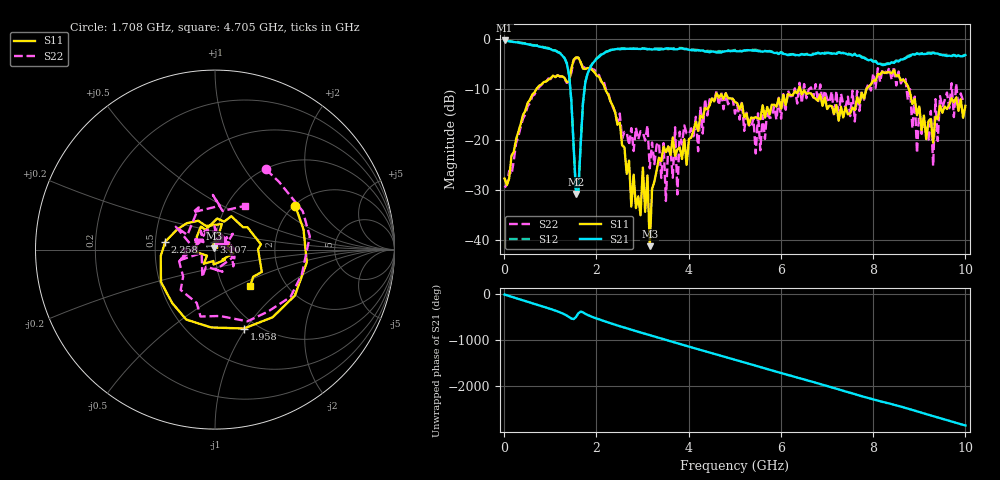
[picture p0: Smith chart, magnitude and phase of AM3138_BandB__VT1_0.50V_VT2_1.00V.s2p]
! Date/Time: Tue, Nov 13, 2018 4:39 PM
! Network Analyzer: Agilent Technologies E8364B Rev: A.07.50.67
! Sweep from 0.010 to 10.000 GHz, 201 Points, Sweep Type: LIN
! Power Supply: 0.500 V, 0.000 A
# Hz S DB R 50
!freq MagS11 AngS11 MagS21 AngS21 MagS12 AngS12 MagS22 AngS22
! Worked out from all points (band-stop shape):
!   201 points, 10 MHz to 10 GHz, reference 50 ohm
!   highest |S21| = -0.24 dB at 10 MHz (marker M1); lowest = -30.9 dB at 1.558 GHz (marker M2)
!   |S21| within 3 dB of the highest: start of sweep to 1.258 GHz; 2.091 GHz to 7.641 GHz (5.55 GHz wide, 114 % of centre)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
!   lowest |S11| = -41.3 dB at 3.157 GHz (marker M3), VSWR 1.02, Z = 49.6 + j0.782 ohm
!   |S11| at or under -10 dB: 2.195 GHz to 6.383 GHz (4.189 GHz wide, 97.7 % of centre); 6.421 GHz to 7.852 GHz (1.431 GHz wide, 20 % of centre); 8.777 GHz to end of sweep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
!   |S22| runs from -32.3 to -3.7 dB; largest |S21 - S12| = 0.028
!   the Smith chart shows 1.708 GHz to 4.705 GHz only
!   S11 on the Smith chart (normalised r, x): 1.708 GHz: 2.03, +1.33; 1.958 GHz: 0.87, -0.98; 2.258 GHz: 0.56, +0.05; 3.107 GHz: 0.98, +0.08; 4.705 GHz: 1.33, -0.60
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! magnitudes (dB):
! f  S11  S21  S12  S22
! 10 MHz  -27.8  -0.2  -0.3  -29.6
! 1.309 GHz  -7.7  -3.8  -3.7  -7.9
! 1.558 GHz  -3.6  -30.9  -30.7  -3.8
! 1.708 GHz  -5.9  -12.8  -12.8  -5.5
! 1.958 GHz  -6.6  -4.4  -4.3  -6.1
! 2.258 GHz  -11.0  -2.4  -2.4  -10.6
! 2.757 GHz  -33.4  -1.9  -1.9  -17.7
! 3.107 GHz  -27.2  -1.9  -2.0  -17.2
! 3.157 GHz  -41.3  -2.0  -1.9  -25.7
! 3.357 GHz  -23.6  -2.1  -1.8  -20.6
! 3.507 GHz  -22.5  -1.8  -1.9  -32.3
! 3.706 GHz  -23.3  -2.0  -1.8  -17.5
! 3.756 GHz  -22.0  -2.0  -1.8  -30.9
! 3.806 GHz  -21.6  -1.8  -1.7  -18.4
! 4.705 GHz  -11.0  -2.6  -2.4  -10.5
! 5.005 GHz  -12.5  -2.3  -2.1  -14.8
! 6.703 GHz  -11.5  -3.0  -2.9  -11.6
! 8.352 GHz  -6.6  -4.9  -4.8  -5.6
! 9.251 GHz  -15.9  -2.9  -2.7  -14.3
! 9.301 GHz  -20.6  -2.7  -2.6  -25.3
! 9.351 GHz  -15.4  -2.8  -2.8  -11.9
! 10 GHz  -13.3  -3.2  -3.1  -12.6
